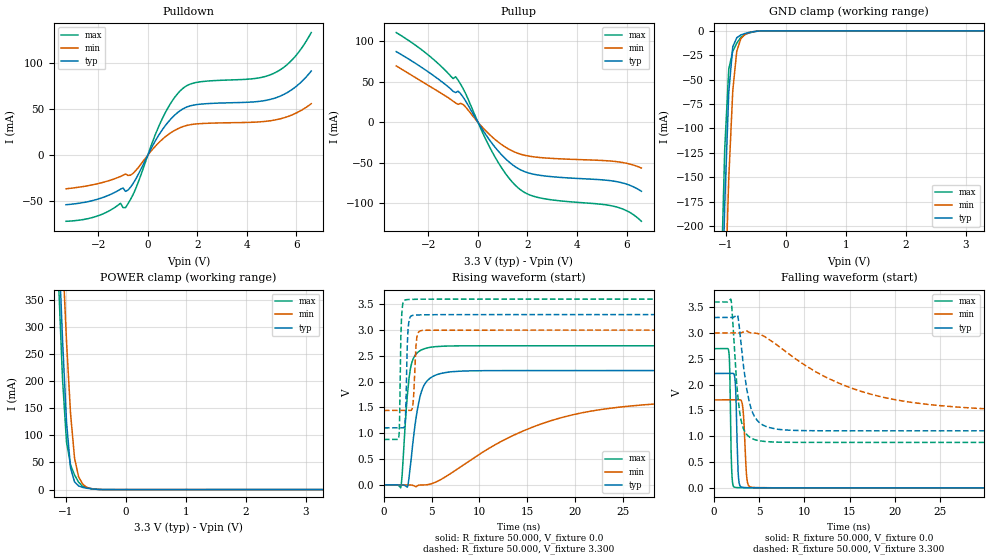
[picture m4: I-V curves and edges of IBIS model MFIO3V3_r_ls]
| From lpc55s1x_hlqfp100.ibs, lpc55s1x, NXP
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|   Model MFIO3V3_r_ls
[Model] MFIO3V3_r_ls
Model_type I/O
Polarity   Non-Inverting
Enable   Active-Low
Vinl =  0.990V
Vinh =  2.310V
Vmeas =  1.650V
Cref =  0.0F
Rref =  100.000
Vref =  0.0V
C_comp   1.906pF   1.877pF   1.925pF
C_comp_pullup   1.141pF   1.113pF   1.145pF
C_comp_pulldown   0.641pF   0.601pF   0.647pF
[Model Spec]
Vinh   2.310V   2.100V   2.520V
Vinl   0.990V   0.900V   1.080V
Vmeas   1.650V   1.500V   1.800V
Vref   0.0V   0.0V   0.0V
Cref   0.0F   0.0F   0.0F
Rref   100.000   100.000   100.000
[Temperature Range]   25.000   0.125k   -40.000
[Voltage Range]   3.300V   3.000V   3.600V
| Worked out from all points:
|   slope of the pulldown table from 0 to 0.495 V, typ, clamps not added: 20.7 ohm
|   slope of the pullup table from 0 to 0.495 V, typ, clamps not added: 21.4 ohm
|   GND clamp passes 1 mA (typ) near -0.56 V on its own axis
|   POWER clamp passes 1 mA (typ) near -0.54 V on its own axis
|   rising waveform, R_fixture 50.000, V_fixture 0.0: 20-80 % time 1.05ns typ, 11.9ns min, 671ps max; typ from 0 V to 2.21 V
|   rising waveform, R_fixture 50.000, V_fixture 3.300: 20-80 % time 177ps typ, 234ps min, 147ps max; typ from 1.1 V to 3.3 V
|   falling waveform, R_fixture 50.000, V_fixture 0.0: 20-80 % time 203ps typ, 281ps min, 162ps max; typ from 2.21 V to 0 V
|   falling waveform, R_fixture 50.000, V_fixture 3.300: 20-80 % time 1.14ns typ, 11.2ns min, 742ps max; typ from 3.3 V to 1.1 V
[Pulldown]
|Voltage   I(typ)   I(min)   I(max)
-3.3V     -53.7mA    -36.43mA   -71.67mA
-2.1V     -48.29mA   -31.37mA   -66.51mA
-1.1V     -36.82mA   -23.05mA   -52.1mA
-900mV    -39.2mA    -20.39mA   -56.91mA
-600mV    -30.96mA   -19.83mA   -42.97mA
600mV     28.07mA    17.5mA     40.4mA
1V        41.17mA    25.53mA    59.41mA
1.4V      49.87mA    30.79mA    72.04mA
2V        54.93mA    33.94mA    79.03mA
5V        60.84mA    37.53mA    87.68mA
5.9V      72.62mA    44.52mA    105.4mA
6.6V      91.19mA    55.78mA    132.9mA
[Pullup]
|Voltage   I(typ)   I(min)   I(max)
-3.3V     87.16mA    69.54mA    110.7mA
-2.1V     64.12mA    47.22mA    85.31mA
-1V       38.1mA     25.85mA    53.88mA
-900mV    36.64mA    23.75mA    56.16mA
-800mV    38.25mA    22.02mA    51.93mA
-600mV    31.06mA    21.93mA    41.58mA
700mV     -31.25mA   -21.55mA   -43.56mA
1.2V      -47.6mA    -32.42mA   -66.97mA
1.7V      -58.52mA   -39.3mA    -83.05mA
2.6V      -66.01mA   -43.88mA   -94.06mA
5.6V      -73.4mA    -48.74mA   -104.7mA
6.6V      -85.32mA   -56.6mA    -122.4mA
[GND_clamp]
|Voltage   I(typ)   I(min)   I(max)
-3.3V     -7.222A    -7.177A    -7.278A
-1.089V   -337.1mA   -440.8mA   -274.1mA
-1.022V   -178.2mA   -284.2mA   -121mA
-955mV    -63.05mA   -151.6mA   -39.25mA
-888mV    -16.33mA   -61.34mA   -20.9mA
-821mV    -7.066mA   -20.84mA   -12.66mA
-754mV    -4.265mA   -8.157mA   -6.693mA
-687mV    -2.794mA   -3.896mA   -3.841mA
-620mV    -1.725mA   -1.894mA   -2.339mA
-419mV    -112.4uA   -138.2uA   -135uA
3.3V      0A         0A         -7.009uA
[POWER_clamp]
|Voltage   I(typ)   I(min)   I(max)
-3.3V     8.016A     7.986A     8.074A
-1.122V   463.7mA    614.3mA    385mA
-1.055V   276.3mA    434.9mA    203.9mA
-988mV    124mA      272.3mA    87.13mA
-921mV    39.96mA    140.1mA    45.6mA
-854mV    14.17mA    57.77mA    27.03mA
-787mV    6.855mA    23.75mA    13.68mA
-720mV    4.075mA    10.22mA    6.123mA
-653mV    2.616mA    4.368mA    3.615mA
-586mV    1.55mA     1.867mA    2.107mA
-452mV    281.1uA    359.9uA    338.7uA
3.3V      0A         0A         7.017uA
[Ramp]
| variable   typ   min   max
dV/dt_r   1.329/1.050n   1.022/11.911n   1.618/0.671n
dV/dt_f   1.317/1.135n   0.935/11.179n   1.632/0.745n
R_load = 50.000
[Rising Waveform]
R_fixture= 50.000
V_fixture= 0.0
V_fixture_min= 0.0
V_fixture_max= 0.0
|time   V(typ)   V(min)   V(max)
0s        11.38nV    124.8nV    46.5nV
1.76ns    11.35uV    -379.5nV   -52.4mV
1.89ns    125.5uV    -254nV     156mV
2.47ns    -34.61mV   65.09uV    1.767V
2.93ns    645.9mV    -4.783mV   2.378V
3.68ns    1.636V     -4.548mV   2.589V
4.97ns    2.087V     21.85mV    2.67V
15.4ns    2.215V     1.107V     2.696V
25.87ns   2.215V     1.53V      2.696V
100ns     2.215V     1.704V     2.696V
[Rising Waveform]
R_fixture= 50.000
V_fixture= 3.300
V_fixture_min= 3.000
V_fixture_max= 3.600
|time   V(typ)   V(min)   V(max)
0s        1.105V     1.442V     880.4mV
1.55ns    1.105V     1.442V     919.2mV
1.84ns    1.105V     1.442V     3.234V
2.22ns    1.223V     1.442V     3.583V
2.38ns    2.203V     1.442V     3.59V
2.68ns    3.223V     1.441V     3.594V
3.05ns    3.286V     1.593V     3.596V
3.45ns    3.293V     2.863V     3.598V
4.04ns    3.296V     2.994V     3.599V
100ns     3.3V       3V         3.6V
[Falling Waveform]
R_fixture= 50.000
V_fixture= 0.0
V_fixture_min= 0.0
V_fixture_max= 0.0
|time   V(typ)   V(min)   V(max)
0s        2.215V     1.704V     2.696V
1.63ns    2.215V     1.704V     2.641V
1.73ns    2.215V     1.704V     2.3V
1.97ns    2.216V     1.704V     265.9mV
2.38ns    1.949V     1.704V     8.551mV
2.68ns    252.6mV    1.704V     4.207mV
3.21ns    8.403mV    1.507V     1.553mV
3.64ns    3.966mV    164.2mV    1.001mV
4.27ns    2.116mV    8.843mV    551.5uV
100ns     15.88nV    209.8nV    49.27nV
[Falling Waveform]
R_fixture= 50.000
V_fixture= 3.300
V_fixture_min= 3.000
V_fixture_max= 3.600
|time   V(typ)   V(min)   V(max)
0s        3.3V       3V         3.6V
1.87ns    3.3V       3V         3.648V
2.61ns    3.334V     3V         1.81V
3.09ns    2.622V     3.009V     1.234V
3.83ns    1.711V     3.015V     996.5mV
4.37ns    1.414V     3.001V     942.3mV
5.1ns     1.252V     2.972V     910mV
14.33ns   1.105V     1.991V     880.4mV
25.13ns   1.105V     1.591V     880.4mV
100ns     1.105V     1.442V     880.4mV
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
